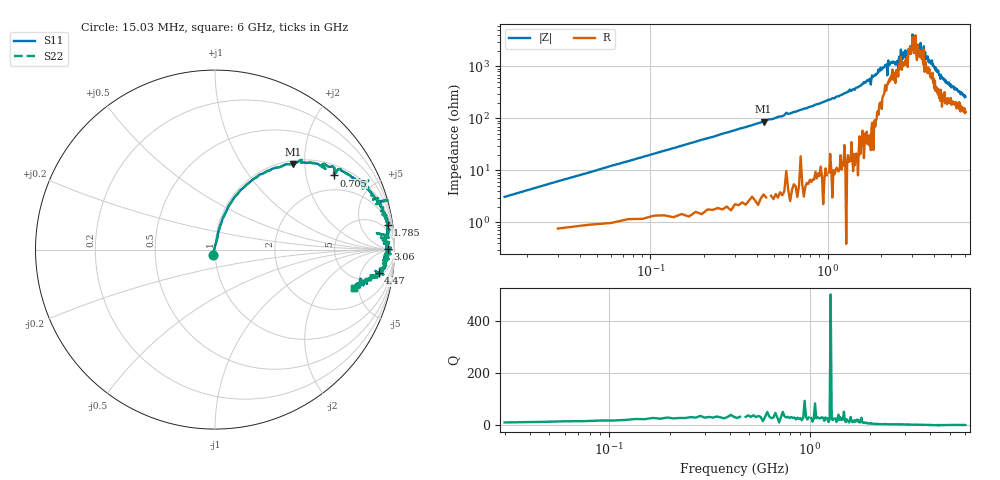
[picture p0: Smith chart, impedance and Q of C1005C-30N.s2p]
!	Network	Analyzer	HP8753E.07.74:	Oct	30	2002	Serial	No.	JP38451487
!	Hewlett-Packard
!	7	Sep	2009	9:02:54
!	Frequency	S11	S21	S12	S22
#	HZ	S	RI	R	50
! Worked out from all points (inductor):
!   400 points, 15.03 MHz to 6 GHz, reference 50 ohm
!   read as one part in series: L = 32.1 nH near 45.03 MHz
!   highest Q = 29.5 at 435 MHz (marker M1), where L = 31.8 nH
!   self-resonance near 3.06 GHz
!   S11 on the Smith chart (normalised r, x): 15.03 MHz: 0.97, -0.06; 705 MHz: 1.37, +2.90; 1.785 GHz: 3, +13; 3.06 GHz: 54, +5; 4.47 GHz: 6, -11; 6 GHz: 3.65, -4.48
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1.502992e7  -0.0126 -0.0293  1.01 0.0293  1.01 0.0293  -0.0126 -0.0293
6.00297e7  0.0239 0.118  0.976 -0.118  0.976 -0.118  0.0239 0.118
1.200294e8  0.0656 0.221  0.934 -0.221  0.934 -0.221  0.0656 0.221
4.350278e8  0.433 0.476  0.567 -0.476  0.567 -0.476  0.433 0.476
7.050265e8  0.662 0.413  0.338 -0.413  0.338 -0.413  0.662 0.413
1.020025e9  0.829 0.357  0.171 -0.357  0.171 -0.357  0.829 0.357
1.785021e9  0.962 0.139  0.0379 -0.139  0.0379 -0.139  0.962 0.139
2.01002e9  0.963 0.105  0.037 -0.105  0.037 -0.105  0.963 0.105
2.505017e9  0.925 0.0676  0.0747 -0.0676  0.0747 -0.0676  0.925 0.0676
2.595017e9  0.966 0.0301  0.0345 -0.0301  0.0345 -0.0301  0.966 0.0301
2.835016e9  0.943 0.0454  0.0569 -0.0454  0.0569 -0.0454  0.943 0.0454
3.015015e9  0.979 0.0103  0.0214 -0.0103  0.0214 -0.0103  0.979 0.0103
3.060015e9  0.964 0.00314  0.0364 -0.00314  0.0364 -0.00314  0.964 0.00314
3.135014e9  0.975 0.00272  0.0246 -0.00272  0.0246 -0.00272  0.975 0.00272
3.195014e9  0.946 -0.0298  0.0537 0.0298  0.0537 0.0298  0.946 -0.0298
3.345013e9  0.975 -0.0234  0.0251 0.0234  0.0251 0.0234  0.975 -0.0234
3.495013e9  0.965 -0.0188  0.0346 0.0188  0.0346 0.0188  0.965 -0.0188
3.525012e9  0.947 -0.0563  0.0527 0.0563  0.0527 0.0563  0.947 -0.0563
4.00501e9  0.952 -0.0878  0.0479 0.0878  0.0479 0.0878  0.952 -0.0878
4.470008e9  0.912 -0.131  0.0885 0.131  0.0885 0.131  0.912 -0.131
5.010005e9  0.866 -0.16  0.134 0.16  0.134 0.16  0.866 -0.16
6e9  0.777 -0.215  0.223 0.215  0.223 0.215  0.777 -0.215
